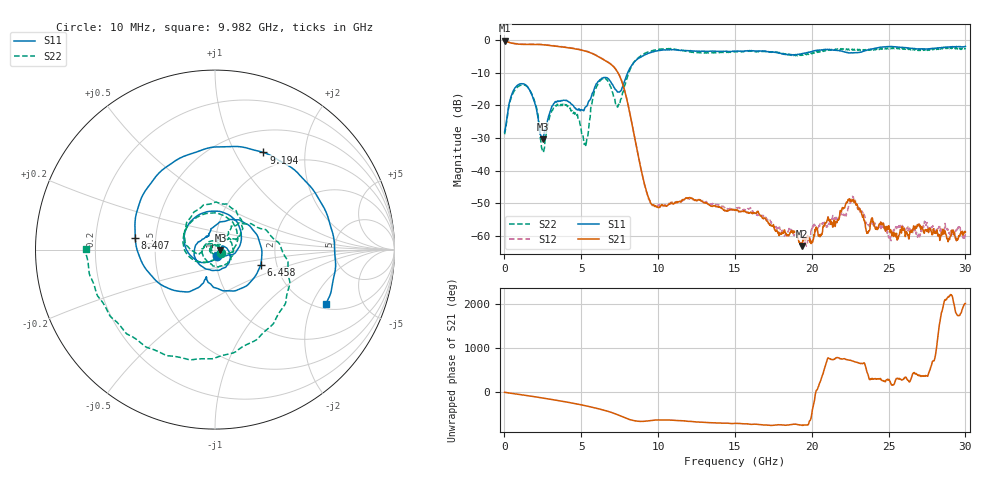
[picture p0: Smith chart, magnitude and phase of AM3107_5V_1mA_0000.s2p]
# Hz S DB R 50.0
!freq dBS11 angS11 dBS21 angS21 dBS12 angS12 dBS22 angS22
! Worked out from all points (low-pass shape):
!   1601 points, 10 MHz to 30 GHz, reference 50 ohm
!   highest |S21| = -0.19 dB at 10 MHz (marker M1); lowest = -63.0 dB at 19.35 GHz (marker M2)
!   |S21| within 3 dB of the highest: start of sweep to 5.143 GHz
!   lowest |S11| = -30.4 dB at 2.484 GHz (marker M3), VSWR 1.06, Z = 53.1 - j0.277 ohm
!   |S11| at or under -10 dB: start of sweep to 8.02 GHz
!   |S22| runs from -34.4 to -2.2 dB; largest |S21 - S12| = 0.012
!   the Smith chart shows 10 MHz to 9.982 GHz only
!   S11 on the Smith chart (normalised r, x): 10 MHz: 1.02, -0.08; 6.458 GHz: 1.65, -0.30; 8.407 GHz: 0.38, +0.06; 9.194 GHz: 0.77, +1.31; 9.982 GHz: 2.23, -2.55
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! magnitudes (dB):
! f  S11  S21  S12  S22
! 10 MHz  -28.1  -0.2  -0.1  -28.8
! 572.3 MHz  -15.6  -1.0  -0.9  -16.1
! 1.341 GHz  -13.6  -1.3  -1.2  -13.8
! 1.997 GHz  -19.6  -1.3  -1.2  -19.3
! 2.484 GHz  -30.4  -1.4  -1.3  -33.8
! 3.421 GHz  -18.7  -1.9  -1.8  -19.7
! 5.015 GHz  -21.3  -3.1  -3.0  -28.3
! 5.314 GHz  -20.3  -3.4  -3.3  -31.8
! 5.858 GHz  -14.6  -4.4  -4.3  -15.6
! 6.458 GHz  -11.4  -6.0  -5.9  -11.5
! 7.376 GHz  -15.9  -9.9  -9.8  -20.4
! 8.407 GHz  -7.0  -28.2  -28.1  -6.8
! 9.194 GHz  -4.4  -45.4  -45.6  -3.9
! 9.982 GHz  -3.3  -51.2  -50.5  -2.8
! 10.02 GHz  -3.2  -51.3  -50.6  -2.9
! 15.01 GHz  -3.4  -52.1  -52.0  -3.5
! 19.35 GHz  -4.2  -63.0  -59.8  -4.4
! 20.01 GHz  -3.4  -62.0  -57.4  -4.1
! 22.52 GHz  -3.9  -49.1  -49.7  -2.8
! 23.65 GHz  -3.0  -59.0  -56.5  -3.1
! 25.01 GHz  -2.0  -56.8  -60.5  -2.6
! 30 GHz  -1.9  -58.7  -59.0  -2.4
